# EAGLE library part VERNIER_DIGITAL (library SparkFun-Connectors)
British Telecom Connector - BTD Digital (female) This device is useful when designing a project that uses any of the analog sensors in the Vernier ecosystem (sensors and/or controllers) SparkFun Products: SparkFun Vernier Interface Shield (DEV-12858) British Telecom Connector - BTD (female) More information about the Vernier ecosystem can be found here: http://www.vernier.com/engineering/arduino/
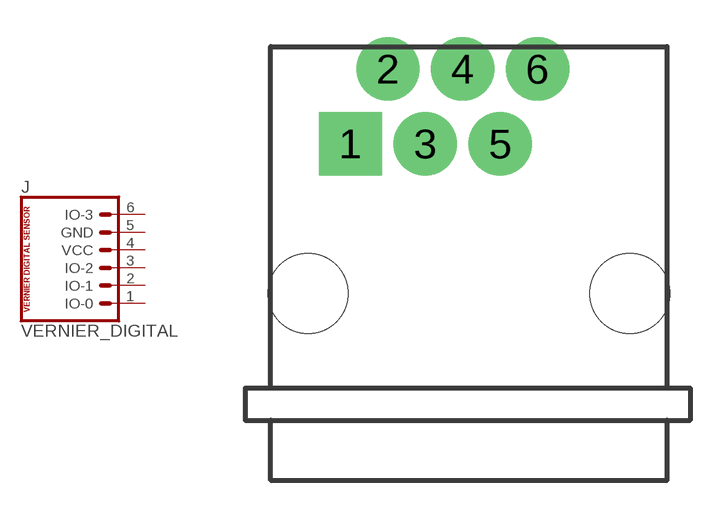
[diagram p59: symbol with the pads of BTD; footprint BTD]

Designator prefix J

## VERNIER_DIGITAL (PROD_ID: CONN-11654; SF_ID: PRT-12754)  [BTD]
1  IO-0  pas
2  IO-1  pas
3  IO-2  pas
4  VCC  pas
5  GND  pas
6  IO-3  pas

## Footprint BTD (pad centres in mm)
British Telecom Connector - Right Angle Female Digital Specifications: Pin count: 6 Datasheet referenced for footprint Example device(s): VERNIER_DIGITAL
drill 1.4 pad 2.54 square: 1 -4.75,6
drill 1.4 pad 2.54: 2 -3.25,9; 3 -1.75,6; 4 -0.25,9; 5 1.25,6; 6 2.75,9
hole 3.2 at 6.45,0
hole 3.2 at -6.45,0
